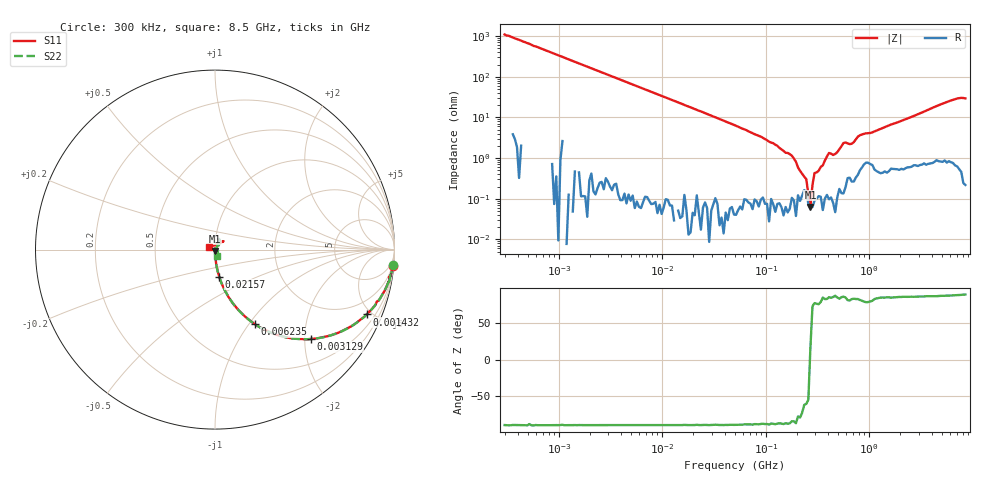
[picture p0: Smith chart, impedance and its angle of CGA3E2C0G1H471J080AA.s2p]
! S-parameter Generated by TDK Corporation
! Copyright(C) 2015 TDK Corporation.
! All Rights Reserved.
! TDK P/N: CGA3E2C0G1H471J080AA (Multilayer Ceramic Chip Capacitors)
! Property: C=470pF
! Size(LxWxT): 1.6x0.8x0.8mm, 0.063x0.031x0.031inches
! Model Type: s2p (Touchstone File Format Version 1.0)
! Frequency: DC=Yes Start=0.3MHz Stop=8500MHz 225points Log-sweep
! Note:
! Model Generated on Jun. 23, 2015
! Hash(MD5):
! Port Assignments:
!  1 ---| |--- 2
! Applicable Conditions:
!  Temperature = 25 degC
!  DC Bias Voltage = 0 V
!  Small Signal Operation
! Terms and conditions regarding TDK Simulation Models
! (1)This simulation model is being provided solely for informational purposes. Please refer to the specifications of the products in terms of detailed characteristics of such products.
! (2)In no event shall TDK Corporation of any of its subsidiaries be liable for any loss or damage arising, directly or indirectly,
!  From any information contained in this simulation model, including, but not limited to loss or damages arising from any inaccuracies, omissions or errors in connection with such information.
! (3)Any and all copyrights on this simulation model are owned by TDK Corporation.
!  Duplication or redistribution of this simulation model without prior written permission from TDK Corporation is prohibited.
! (4)This simulation model is subject to any modification or change without any prior notice.
! (5)Neither TDK Corporation nor any of its subsidiaries shall make any warranty, express or implied,
!  Including but not limited to the correctness, implied warranties of merchantability and fitness for a particular purpose with respect to this simulation models.
! (6)The use of this simulation model shall be deemed to have consented to the terms and conditions hereof.
# MHz S MA R 50
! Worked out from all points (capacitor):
!   224 points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, 300 kHz to 8.5 GHz, reference 50 ohm
!   read as one part in series: C = 477 pF near 314.1 kHz
!   lowest |Z| = 63 mohm at 270.4 MHz (marker M1)
!   series resonance near 268.6 MHz, so ESL is about 740 pH
!   S11 on the Smith chart (normalised r, x): 300 kHz: 1, -22; 1.432 MHz: 1.01, -4.67; 3.129 MHz: 1.00, -2.13; 6.235 MHz: 1.00, -1.07; 21.57 MHz: 1.00, -0.31; 8.5 GHz: 0.93, +0.03
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0.3  0.9959 -5.2  0.09093 84.8  0.09093 85.1  0.9959 -4.9
1.432013  0.9183 -23.1  0.3943 66.7  0.3939 66.8  0.9187 -23.2
1.72111  0.8885 -27.3  0.4584 62.7  0.4578 62.7  0.8885 -27.3
3.12867  0.729 -43.1  0.6834 46.8  0.683 46.8  0.7294 -43.1
6.235074  0.472 -61.8  0.8804 28.1  0.8815 28.1  0.4718 -61.9
9.430415  0.3338 -70.4  0.9424 19.4  0.9419 19.4  0.3333 -70.6
21.57293  0.1525 -81.1  0.9862 8.6  0.9868 8.6  0.1519 -81.2
51.67171  0.06369 -86.0  0.9972 3.5  0.9978 3.4  0.06353 -86.4
270.4017  0.00786 -83.7  0.9991 -0.4  0.9994 -0.4  0.006689 -90.3
283.1228  0.006808 -83.0  0.9994 -0.6  0.9991 -0.6  0.006104 -88.7
356.2888  0.003484 -72.9  0.9997 -0.9  0.9987 -0.9  0.002361 -103.8
408.9767  0.0009658 -34.9  0.998 -1.6  0.999 -1.5  0.0003854 -75.6
448.3627  0.001547 -25.7  0.9977 -1.4  0.9997 -1.3  0.001253 130.4
564.2308  0.003433 55.9  0.997 -2.5  0.9987 -2.4  0.005195 94.0
710.042  0.006257 50.5  0.9973 -2.6  0.9962 -2.5  0.004257 81.5
853.3868  0.009462 58.1  0.9939 -3.9  0.994 -3.9  0.01051 43.8
1551.304  0.00812 64.1  0.9948 -6.9  0.9943 -6.8  0.009295 45.0
2572.272  0.01195 56.4  0.9939 -11.4  0.9928 -11.3  0.01168 40.0
5884.306  0.06189 46.8  0.9884 -26.1  0.9873 -26.0  0.06044 67.3
7404.957  0.05922 47.4  0.9895 -32.6  0.9877 -32.6  0.055 62.8
8118.083  0.02612 84.5  0.9918 -35.5  0.9911 -35.4  0.0197 22.3
8500  0.03731 158.7  0.9909 -37.0  0.9919 -37.0  0.03908 -70.5
